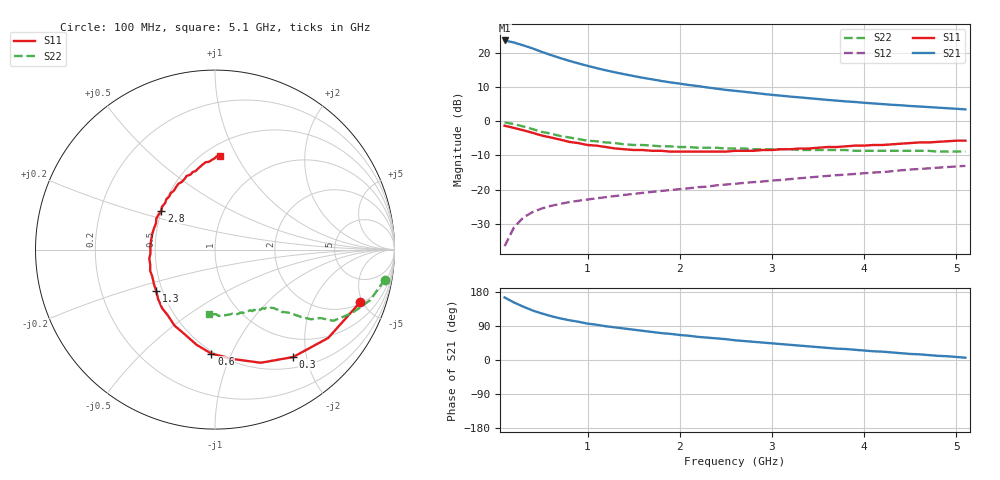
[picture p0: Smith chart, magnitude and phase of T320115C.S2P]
!AT-32011
!S PARAMETERS at Vce=5  V  Ic=5mA.  LAST UPDATED 01-05-95
# ghz s ma r 50
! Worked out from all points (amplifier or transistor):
!   51 points, 100 MHz to 5.1 GHz, reference 50 ohm
!   highest |S21| = 23.6 dB at 100 MHz (marker M1)
!   |S21| within 3 dB of that: start of sweep to 469.3 MHz
!   unconditionally stable (mu >= 1): 1.867 GHz to 4.948 GHz
!   at 900 MHz: K = 0.64, MSG = 20.1 dB, |S12| = -23.2 dB
!   at 2.6 GHz: K = 1.09, MAG = 11.7 dB, |S12| = -18.3 dB
!   at 5.1 GHz: K = 1.00, MSG = 8.2 dB, |S12| = -13.0 dB
!   S11 on the Smith chart (normalised r, x): 100 MHz: 2.11, -4.77; 300 MHz: 0.67, -1.77; 600 MHz: 0.48, -0.84; 1.3 GHz: 0.46, -0.25; 2.8 GHz: 0.50, +0.25; 5.1 GHz: 0.60, +0.85
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0.1  0.86 -20.0  15.11 165.0  0.015 79.0  0.96 -10.0
0.2  0.8 -38.0  14.11 152.0  0.028 70.0  0.91 -18.0
0.3  0.74 -54.0  12.85 141.0  0.039 63.0  0.84 -25.0
0.4  0.68 -68.0  11.6 131.0  0.047 58.0  0.77 -31.0
0.5  0.62 -80.0  10.32 123.0  0.053 54.0  0.7 -33.0
0.6  0.58 -92.0  9.27 116.0  0.058 51.0  0.66 -36.0
0.7  0.54 -101.0  8.39 110.0  0.062 49.0  0.61 -38.0
0.8  0.5 -110.0  7.63 105.0  0.066 48.0  0.58 -39.0
1  0.45 -126.0  6.44 96.0  0.072 46.0  0.52 -42.0
1.2  0.42 -139.0  5.53 89.0  0.078 46.0  0.49 -43.0
1.3  0.4 -145.0  5.17 86.0  0.081 46.0  0.48 -44.0
1.5  0.38 -157.0  4.57 80.0  0.087 46.0  0.45 -46.0
1.8  0.37 -172.0  3.87 71.0  0.096 46.0  0.43 -49.0
2.2  0.36 168.0  3.26 61.0  0.109 46.0  0.41 -54.0
2.5  0.36 156.0  2.87 55.0  0.119 45.0  0.4 -57.0
2.6  0.37 152.0  2.78 52.0  0.122 45.0  0.4 -58.0
2.8  0.37 144.0  2.6 48.0  0.129 45.0  0.39 -60.0
3.1  0.39 134.0  2.36 42.0  0.139 44.0  0.39 -64.0
3.5  0.41 122.0  2.11 34.0  0.155 43.0  0.38 -69.0
3.7  0.42 116.0  2 30.0  0.163 42.0  0.38 -72.0
4.3  0.46 102.0  1.74 20.0  0.186 40.0  0.37 -80.0
5.1  0.52 87.0  1.49 6.0  0.223 34.0  0.36 -95.0
